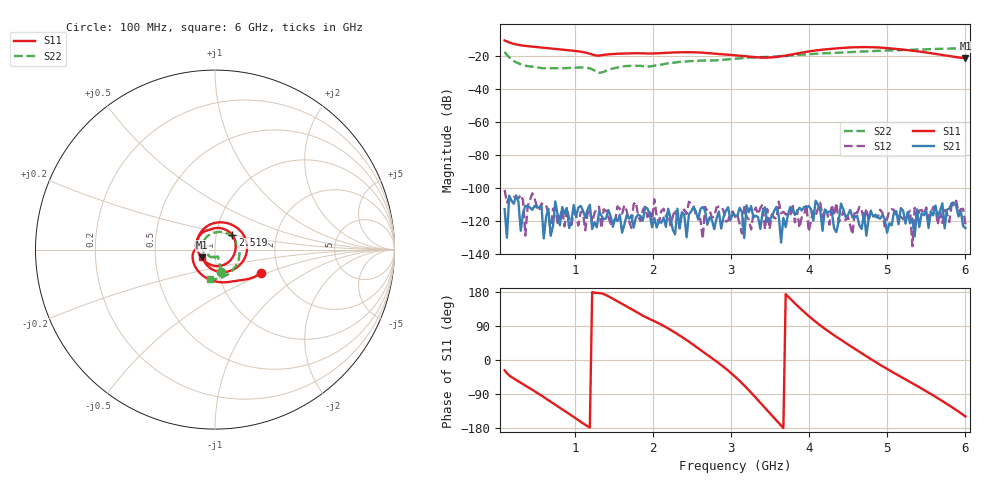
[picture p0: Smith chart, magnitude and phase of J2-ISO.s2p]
!Agilent Technologies,E8364B,MY43040379,A.07.50.67
!Agilent E8364B: A.07.50.67
!Date: Tuesday, March 24, 2026 11:05:04
!Correction: S11(Full 2 Port(1,2))
!S21(Full 2 Port(1,2))
!S12(Full 2 Port(1,2))
!S22(Full 2 Port(1,2))
!S2P File: Measurements: S11, S21, S12, S22:
# Hz S  dB  R 50
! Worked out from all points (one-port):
!   201 points, 100 MHz to 6 GHz, reference 50 ohm
!   lowest |S11| = -21.6 dB at 6 GHz (marker M1), VSWR 1.18, Z = 43.2 - j3.73 ohm
!   |S11| at or under -10 dB: start of sweep to end of sweep
!   S11 on the Smith chart (normalised r, x): 100 MHz: 1.60, -0.46; 2.519 GHz: 1.20, +0.20; 6 GHz: 0.86, -0.07
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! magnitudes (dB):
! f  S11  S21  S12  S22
! 100 MHz  -10.9  -113.1  -101.5  -17.8
! 159 MHz  -12.0  -105.0  -106.3  -21.1
! 218 MHz  -12.9  -109.9  -105.8  -23.3
! 365.5 MHz  -14.2  -111.1  -129.2  -26.2
! 601.5 MHz  -15.3  -130.9  -110.8  -27.7
! 1.103 GHz  -17.9  -114.0  -114.7  -27.2
! 1.192 GHz  -18.9  -110.5  -113.9  -27.8
! 1.31 GHz  -20.0  -114.6  -111.6  -30.4
! 1.634 GHz  -18.8  -122.3  -110.8  -26.5
! 1.811 GHz  -18.6  -116.4  -117.5  -26.2
! 1.929 GHz  -18.8  -112.7  -117.9  -26.7
! 2.076 GHz  -18.6  -120.4  -121.0  -25.8
! 2.342 GHz  -18.1  -124.5  -124.8  -23.9
! 2.519 GHz  -18.0  -111.8  -111.3  -23.3
! 3.05 GHz  -19.8  -116.9  -117.8  -21.9
! 3.374 GHz  -21.2  -125.1  -112.3  -21.0
! 3.522 GHz  -21.1  -117.6  -116.3  -20.8
! 4.053 GHz  -17.1  -120.1  -114.4  -19.0
! 4.584 GHz  -15.0  -118.1  -113.9  -17.8
! 5.027 GHz  -15.6  -121.7  -114.0  -16.9
! 5.41 GHz  -17.6  -123.9  -113.9  -16.4
! 6 GHz  -21.6  -124.6  -122.2  -15.6
